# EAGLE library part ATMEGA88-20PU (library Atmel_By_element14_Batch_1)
8-bit Microcontroller with In-System Programmable Flash
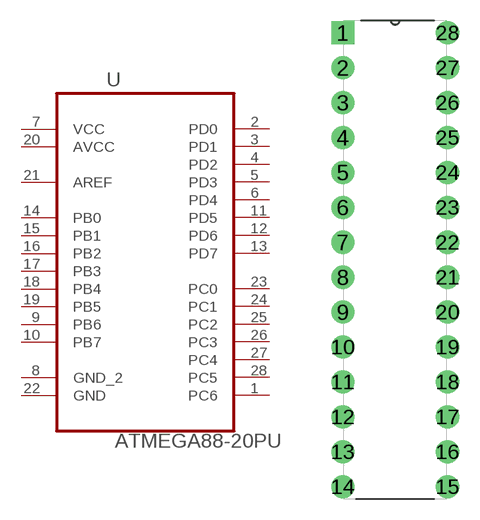
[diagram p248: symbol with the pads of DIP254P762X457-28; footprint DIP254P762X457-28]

Designator prefix U

## ATMEGA88-20PU (MPN: ATMEGA88-20PU; OC_FARNELL: 9171495; OC_NEWARK: 01M6913; PACKAGE: DIP-28; SUPPLIER: Atmel)  [DIP254P762X457-28]
1  PC6  pas
2  PD0  pas
3  PD1  pas
4  PD2  pas
5  PD3  pas
6  PD4  pas
7  VCC  pas
8  GND_2  pas
9  PB6  pas
10  PB7  pas
11  PD5  pas
12  PD6  pas
13  PD7  pas
14  PB0  pas
15  PB1  pas
16  PB2  pas
17  PB3  pas
18  PB4  pas
19  PB5  pas
20  AVCC  pas
21  AREF  pas
22  GND  pas
23  PC0  pas
24  PC1  pas
25  PC2  pas
26  PC3  pas
27  PC4  pas
28  PC5  pas

## Footprint DIP254P762X457-28 (pad centres in mm)
drill 1.118 square: 1 -7.62,33.02
drill 1.118: 2 -7.62,30.48; 3 -7.62,27.94; 4 -7.62,25.4; 5 -7.62,22.86; 6 -7.62,20.32; 7 -7.62,17.78; 8 -7.62,15.24; 9 -7.62,12.7; 10 -7.62,10.16; 11 -7.62,7.62; 12 -7.62,5.08; 13 -7.62,2.54; 14 -7.62,0; 15 0,0; 16 0,2.54; 17 0,5.08; 18 0,7.62; 19 0,10.16; 20 0,12.7; 21 0,15.24; 22 0,17.78; 23 0,20.32; 24 0,22.86; 25 0,25.4; 26 0,27.94; 27 0,30.48; 28 0,33.02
